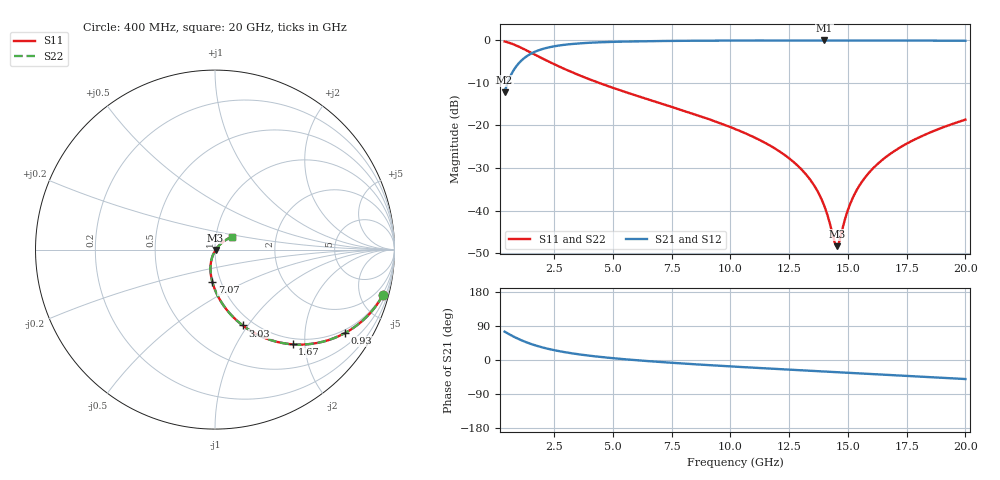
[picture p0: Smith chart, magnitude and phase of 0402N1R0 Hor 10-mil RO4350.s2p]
# MHz S  dB  R 50
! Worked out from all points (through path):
!   1961 points, 400 MHz to 20 GHz, reference 50 ohm
!   highest |S21| = -0.04 dB at 14 GHz (marker M1); lowest = -12.2 dB at 400 MHz (marker M2)
!   lowest |S11| = -48.3 dB at 14.53 GHz (marker M3), VSWR 1.01, Z = 50.3 - j0.213 ohm
!   |S11| at or under -10 dB: 4.419 GHz to end of sweep
!   |S22| runs from -48.3 to -0.3 dB; largest |S21 - S12| = 0
!   S11 on the Smith chart (normalised r, x): 400 MHz: 0.89, -7.41; 930 MHz: 0.89, -3.18; 1.67 GHz: 0.89, -1.76; 3.03 GHz: 0.89, -0.95; 7.07 GHz: 0.91, -0.34; 20 GHz: 1.19, +0.17
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400  -0.27 -15.2  -12.18 74.8  -12.18 74.8  -0.27 -15.2
930  -1.31 -32.7  -5.87 57.3  -5.87 57.3  -1.31 -32.7
1670  -3.31 -50.6  -2.74 39.3  -2.74 39.3  -3.31 -50.6
2300  -5.06 -61.1  -1.64 28.7  -1.64 28.7  -5.06 -61.1
3030  -6.93 -69.9  -1.00 19.9  -1.00 19.9  -6.93 -69.9
3670  -8.42 -75.7  -0.69 14.0  -0.69 14.0  -8.42 -75.7
6940  -14.64 -94.2  -0.17 -4.9  -0.17 -4.9  -14.64 -94.2
7070  -14.87 -94.7  -0.17 -5.5  -0.17 -5.5  -14.87 -94.7
10200  -20.80 -105.7  -0.07 -17.6  -0.07 -17.6  -20.80 -105.7
12220  -26.56 -110.4  -0.04 -24.5  -0.04 -24.5  -26.56 -110.4
12920  -29.71 -110.7  -0.04 -26.8  -0.04 -26.8  -29.71 -110.7
13470  -33.28 -109.0  -0.04 -28.6  -0.04 -28.6  -33.28 -109.0
14000  -38.90 -101.2  -0.04 -30.4  -0.04 -30.4  -38.90 -101.2
14430  -47.23 -60.6  -0.04 -31.8  -0.04 -31.8  -47.23 -60.6
14530  -48.33 -33.4  -0.04 -32.1  -0.04 -32.1  -48.33 -33.4
14640  -47.13 -3.7  -0.04 -32.5  -0.04 -32.5  -47.13 -3.7
15050  -39.10 35.4  -0.04 -33.8  -0.04 -33.8  -39.10 35.4
15410  -34.85 42.2  -0.04 -35.0  -0.04 -35.0  -34.85 42.2
15980  -30.59 45.1  -0.05 -36.9  -0.05 -36.9  -30.59 45.1
16740  -26.91 45.2  -0.05 -39.4  -0.05 -39.4  -26.91 45.2
18140  -22.50 42.5  -0.07 -44.0  -0.07 -44.0  -22.50 42.5
20000  -18.62 37.3  -0.11 -50.2  -0.11 -50.2  -18.62 37.3
